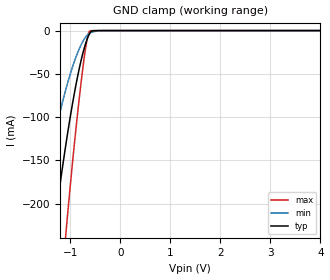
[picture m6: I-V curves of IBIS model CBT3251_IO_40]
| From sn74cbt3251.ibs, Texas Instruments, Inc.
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[Model]   CBT3251_IO_40
Model_type  Terminator
| variable   typ   min   max
C_comp   23.63pF   20.09pF   26.18pF
| C_tri-state   23.63pF   20.09pF   26.18pF
[Temperature Range]   40   100   -40
| Ambient temperature   25   85   -40
[Voltage range]   4   4   4
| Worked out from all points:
|   GND clamp passes 1 mA (typ) near -0.58 V on its own axis
[GND Clamp]
| CBT3251_IO_40
|   Voltage   I(typ)   I(min)   I(max)
-4V       -1.785A    -1.159A    -2.741A
-1.725V   -422mA     -241.7mA   -705.1mA
-1.68V    -399.1mA   -227.5mA   -669.2mA
-1.33V    -232.5mA   -126mA     -402.7mA
-1.1V     -137.1mA   -70.89mA   -244mA
-1.065V   -123.9mA   -63.51mA   -221.4mA
-900mV    -67.55mA   -33.06mA   -122.1mA
-745mV    -25.99mA   -12.41mA   -42.7mA
-665mV    -10.62mA   -5.609mA   -11.13mA
-630mV    -5.664mA   -3.632mA   -2.414mA
-600mV    -2.48mA    -2.39mA    -287uA
4V        2.459nA    3.726nA    2.364nA
